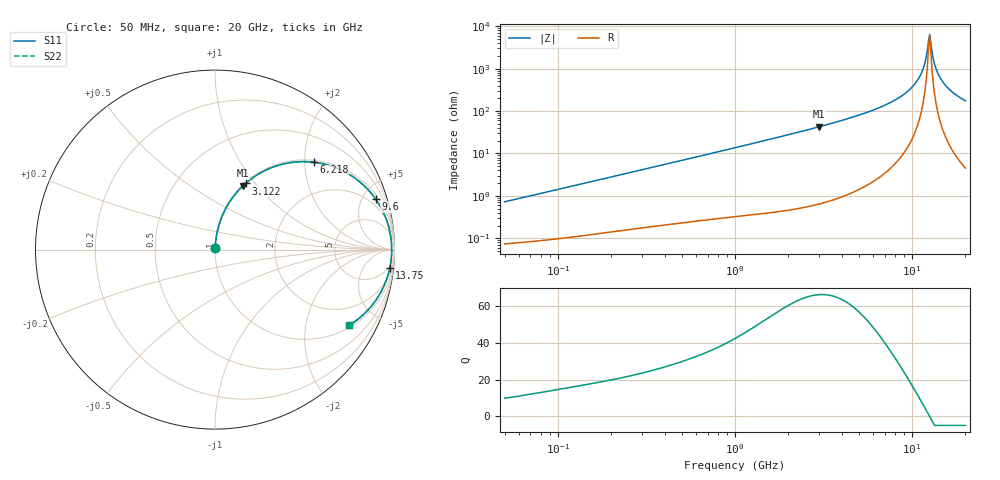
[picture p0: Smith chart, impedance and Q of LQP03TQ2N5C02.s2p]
!Murata Part Number: LQP03TQ2N5C02
!These Parameters are Measured in Series Mode Connection
!  o--[Z]--o
!Port1  Port2
!  o-------o
!Freq. Start=50[MHz] Stop=20[GHz], 401[Steps]
# Hz S RI R 50
!Freq.(Hz) S11(Real) S11(Imag) S21(Real) S21(Imag) S12(Real) S12(Imag) S22(Real) S22(Imag)
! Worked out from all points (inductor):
!   401 points, 50 MHz to 20 GHz, reference 50 ohm
!   read as one part in series: L = 2.28 nH near 51.52 MHz
!   highest Q = 66.2 at 2.985 GHz (marker M1), where L = 2.27 nH
!   self-resonance near 12.38 GHz
!   S11 on the Smith chart (normalised r, x): 50 MHz: 1.00, +0.01; 3.122 GHz: 1.01, +0.90; 6.218 GHz: 1.05, +2.22; 9.6 GHz: 1.32, +6.20; 13.75 GHz: 4, -18; 20 GHz: 1.09, -3.49
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5e7  0.000788 0.0072  0.9992 -0.0072  0.9992 -0.0072  0.000788 0.0072
1.364002e8  0.00151 0.0192  0.9985 -0.0192  0.9985 -0.0192  0.00151 0.0192
3.721004e8  0.00458 0.0509  0.9954 -0.0509  0.9954 -0.0509  0.00458 0.0509
1e9  0.0213 0.133  0.9787 -0.133  0.9787 -0.133  0.0213 0.133
2.728004e9  0.1331 0.3322  0.8669 -0.3322  0.8669 -0.3322  0.1331 0.3322
2.98453e9  0.1572 0.3566  0.8428 -0.3566  0.8428 -0.3566  0.1572 0.3566
3.121702e9  0.1708 0.3689  0.8292 -0.3689  0.8292 -0.3689  0.1708 0.3689
4.405649e9  0.3164 0.457  0.6836 -0.457  0.6836 -0.457  0.3164 0.457
6.217679e9  0.55 0.4869  0.45 -0.4869  0.45 -0.4869  0.55 0.4869
7.442007e9  0.6992 0.4451  0.3008 -0.4451  0.3008 -0.4451  0.6992 0.4451
9.600142e9  0.8943 0.2829  0.1057 -0.2829  0.1057 -0.2829  0.8943 0.2829
1.050288e10  0.943 0.1971  0.057 -0.1971  0.057 -0.1971  0.943 0.1971
1.115139e10  0.9659 0.1337  0.0341 -0.1337  0.0341 -0.1337  0.9659 0.1337
1.166392e10  0.9773 0.0838  0.0227 -0.0838  0.0227 -0.0838  0.9773 0.0838
1.238412e10  0.9844 0.0156  0.0156 -0.0156  0.0156 -0.0156  0.9844 0.0156
1.257102e10  0.9847 -0.0016  0.0153 0.0016  0.0153 0.0016  0.9847 -0.0016
1.276073e10  0.9844 -0.0188  0.0156 0.0188  0.0156 0.0188  0.9844 -0.0188
1.334722e10  0.9798 -0.0701  0.0202 0.0701  0.0202 0.0701  0.9798 -0.0701
1.375312e10  0.9738 -0.1038  0.0262 0.1038  0.0262 0.1038  0.9738 -0.1038
1.460232e10  0.955 -0.1691  0.045 0.1691  0.045 0.1691  0.955 -0.1691
1.573793e10  0.92 -0.2448  0.08 0.2448  0.08 0.2448  0.92 -0.2448
2e10  0.7479 -0.4215  0.2521 0.4215  0.2521 0.4215  0.7479 -0.4215
